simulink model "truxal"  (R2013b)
settings: Solver=ode45  StartTime=0.0  StopTime=10.0  RelTol=1e-3
undefined symbols (not defined in the file): den_s, den_z, K, num_s, num_z, Ts

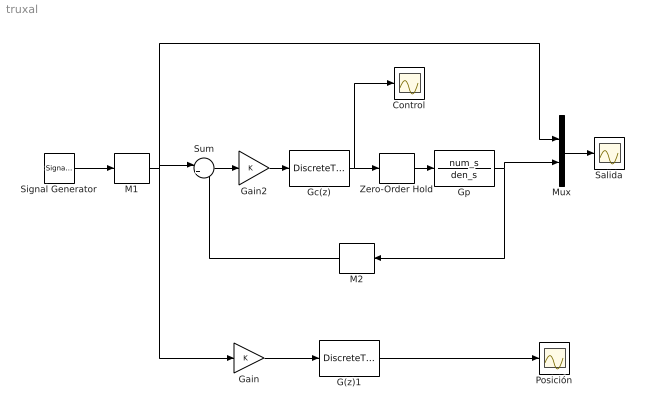
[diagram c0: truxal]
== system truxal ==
  Control : Scope
  G(z)1 : DiscreteTransferFcn  Numerator=num_z  Denominator=den_z  SampleTime=Ts
  Gain : Gain  SampleTime=Ts
  Gain2 : Gain  Gain=K  SampleTime=Ts
  Gc(z) : DiscreteTransferFcn  Numerator=num_z  Denominator=den_z  SampleTime=Ts
  Gp : TransferFcn  Numerator=num_s  Denominator=den_s
  M1 : DiscreteTransferFcn  Numerator=1  Denominator=1  SampleTime=0.01
  M2 : DiscreteTransferFcn  Numerator=1  Denominator=1  SampleTime=Ts
  Mux : Mux  Inputs=2
  Posición : Scope
  Salida : Scope
  Signal Generator : SignalGenerator  WaveForm=square  Frequency=0.3
  Sum : Sum  Inputs=|+-
  Zero-Order Hold : ZeroOrderHold  SampleTime=Ts
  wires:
  Sum/1 -> Gain2/1
  Gp/1 -> Mux/2, M2/1
  G(z)1/1 -> Posición/1
  Mux/1 -> Salida/1
  Gain/1 -> G(z)1/1
  M1/1 -> Sum/1, Gain/1, Mux/1
  Gain2/1 -> Gc(z)/1
  Gc(z)/1 -> Zero-Order Hold/1, Control/1
  Zero-Order Hold/1 -> Gp/1
  M2/1 -> Sum/2
  Signal Generator/1 -> M1/1
